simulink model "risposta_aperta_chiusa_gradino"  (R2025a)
settings: Solver=VariableStepAuto  StartTime=0.0  StopTime=10  RelTol=1e-3
undefined symbols (not defined in the file): denGs, numGs

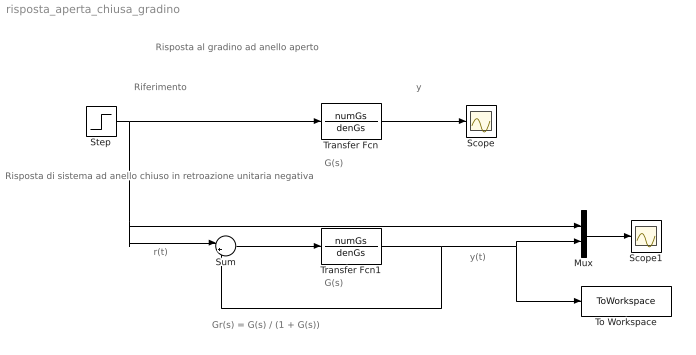
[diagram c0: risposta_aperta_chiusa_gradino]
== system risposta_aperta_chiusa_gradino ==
  note: y(t)
  note: r(t)
  note: Gr(s) = G(s) / (1 + G(s))
  note: y
  note: Riferimento
  note: Risposta di sistema ad anello chiuso in retroazione unitaria negativa
  note: Risposta al gradino ad anello aperto
  note: G(s)
  note: G(s)
  Mux : Mux  Inputs=2
  Scope : Scope
  Scope1 : Scope
  Step : Step  Time=0  SampleTime=0
  Sum : Sum  Inputs=|+-
  To Workspace : ToWorkspace  VariableName=ync  SampleTime=-1
  Transfer Fcn : TransferFcn  Numerator=numGs  Denominator=denGs
  Transfer Fcn1 : TransferFcn  Numerator=numGs  Denominator=denGs
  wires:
  Step/1 -> Sum/1, Mux/1, Transfer Fcn/1
  Transfer Fcn/1 -> Scope/1
  Sum/1 -> Transfer Fcn1/1
  Transfer Fcn1/1 -> To Workspace/1, Mux/2, Sum/2
  Mux/1 -> Scope1/1
